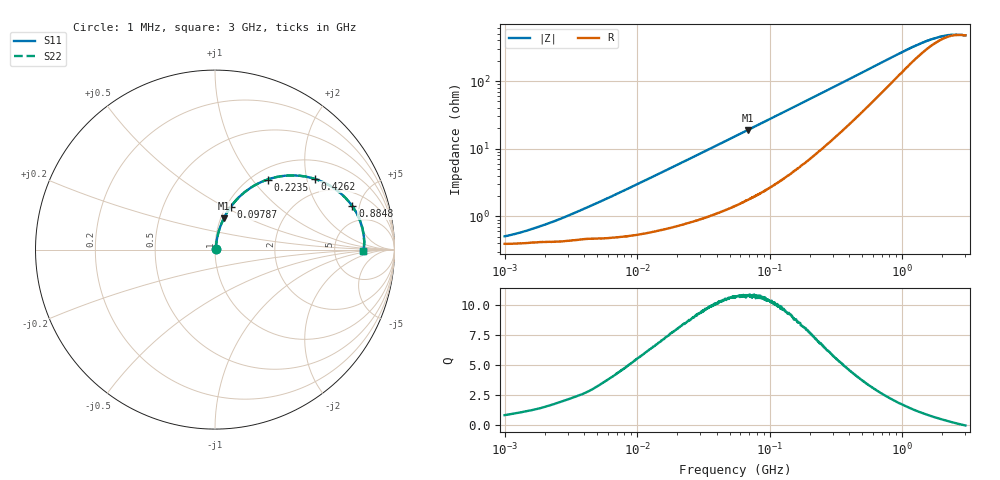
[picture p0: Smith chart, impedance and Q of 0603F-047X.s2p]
!s-Parameter Generated by FASTRON Sdn. Bhd.
!FASTRON P/N : 0603F-047X
!Keysight Technologies: E4991B_MY54100416_A.01.15
!Date: Thu Jun 20 13:01:47 2024
!Version  :Rev00  Thu Jun 20 13:01:47 2024
!Data & Calibration Information:
!Freq  S11  S21  S12  S22
!PortZ  Port1:50+j0  Port2:50+j0
!When reading reference impedance value at option line is always used.
! Remarks : This data is being provided solely for informational purposes.
# Hz S dB R 50
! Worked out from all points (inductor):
!   1601 points, 1 MHz to 3 GHz, reference 50 ohm
!   read as one part in series: L = 47.9 nH near 4.647 MHz
!   highest Q = 10.8 at 68.26 MHz (marker M1), where L = 43.8 nH
!   self-resonance near 2.893 GHz
!   S11 on the Smith chart (normalised r, x): 1 MHz: 1.01, +0.01; 97.87 MHz: 1.05, +0.54; 223.5 MHz: 1.17, +1.20; 426.2 MHz: 1.52, +2.23; 884.8 MHz: 3.14, +4.26; 3 GHz: 10, -0
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1000000  -45.90 39.1  -0.03 -0.2  -0.03 -0.2  -45.90 39.1
1215500  -45.20 44.2  -0.03 -0.2  -0.03 -0.2  -45.20 44.2
1716745  -43.40 52.3  -0.04 -0.3  -0.04 -0.3  -43.40 52.3
2341230  -41.50 59.5  -0.04 -0.4  -0.04 -0.4  -41.50 59.5
3804036  -38.10 67.8  -0.04 -0.7  -0.04 -0.7  -38.10 67.8
1.447069e7  -27.50 79.3  -0.06 -2.4  -0.06 -2.4  -27.50 79.3
3.00453e7  -21.50 79.1  -0.11 -4.8  -0.11 -4.8  -21.50 79.1
5.504702e7  -16.50 76.1  -0.22 -8.6  -0.22 -8.6  -16.50 76.1
6.826239e7  -14.80 74.2  -0.30 -10.5  -0.30 -10.5  -14.80 74.2
9.787053e7  -11.90 69.9  -0.51 -14.6  -0.51 -14.6  -11.90 69.9
1.445978e8  -9.03 63.2  -0.94 -20.6  -0.94 -20.6  -9.03 63.2
2.083556e8  -6.64 54.9  -1.67 -27.5  -1.67 -27.5  -6.64 54.9
2.234756e8  -6.23 53.1  -1.85 -28.9  -1.85 -28.9  -6.23 53.1
3.10929e8  -4.54 44.2  -3.00 -35.7  -3.00 -35.7  -4.54 44.2
4.261603e8  -3.34 35.4  -4.52 -41.5  -4.52 -41.5  -3.34 35.4
5.81181e8  -2.53 27.1  -6.41 -45.5  -6.41 -45.5  -2.53 27.1
7.925923e8  -2.03 19.8  -8.62 -46.4  -8.62 -46.4  -2.03 19.8
8.848309e8  -1.91 17.5  -9.45 -45.8  -9.45 -45.8  -1.91 17.5
1.430499e9  -1.63 9.0  -13.00 -35.5  -13.00 -35.5  -1.63 9.0
1.837163e9  -1.60 5.5  -14.50 -24.8  -14.50 -24.8  -1.60 5.5
2.312676e9  -1.60 2.6  -15.30 -12.4  -15.30 -12.4  -1.60 2.6
3e9  -1.66 -0.4  -15.20 1.8  -15.20 1.8  -1.66 -0.4
